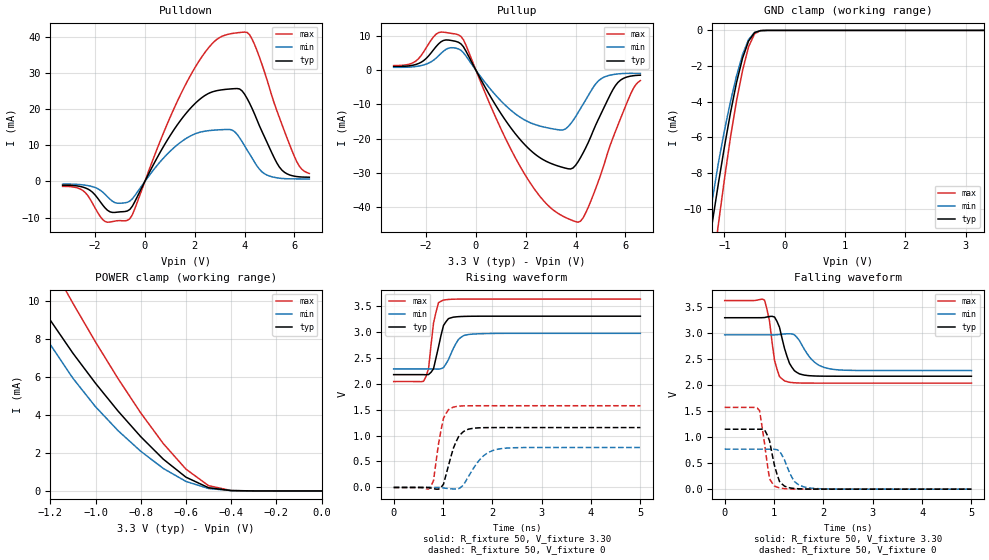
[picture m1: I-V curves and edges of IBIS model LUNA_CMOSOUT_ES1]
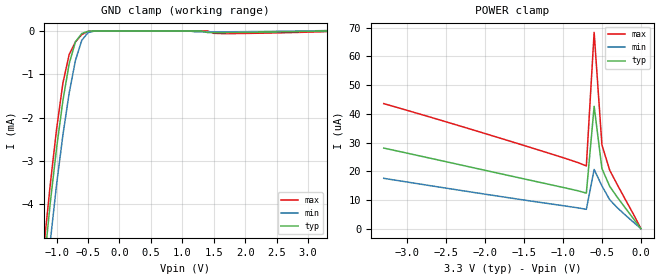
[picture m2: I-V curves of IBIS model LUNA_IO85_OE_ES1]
[IBIS Ver]   3.2
[Comment Char]   |_char
[File name]   sg-9101cx_33v_a.ibs
[File Rev]   1.0
[Date]   2017/11/24 15:54:02
[Source]
[Notes]
[Disclaimer]
This information is for modeling purposes only, and is not guaranteed.
Property of SEIKO EPSON Corp.,
unauthorized reproduction and/or distribution is strictly prohibited.
[Copyright]
Copyright 2017, SEIKO EPSON Corp.
[Component]   SG-9101CA
Si_location Pin
Timing_location Pin
[Manufacturer]   SEIKO EPSON Corp.
| 7050 PKG
| 7050 PKG
[Package]
R_pkg   224m   NA   NA
L_pkg   5.5n   NA   NA
C_pkg   0.144p   NA   NA
[Pin] signal_name   model_name
1   OE   LUNA_IO85_OE_ES1
2   VSS   GND
3   OUT   LUNA_CMOSOUT_ES1
4   VDD   POWER
[Component]   SG-9101CB
Si_location Pin
Timing_location Pin
[Manufacturer]   SEIKO EPSON Corp.
| 5032 PKG
| 5032 PKG
[Package]
R_pkg   200m   NA   NA
L_pkg   2.16n   NA   NA
C_pkg   1.23p   NA   NA
[Pin] signal_name   model_name
1   OE   LUNA_IO85_OE_ES1
2   VSS   GND
3   OUT   LUNA_CMOSOUT_ES1
4   VDD   POWER
[Component]   SG-9101CE
Si_location Pin
Timing_location Pin
[Manufacturer]   SEIKO EPSON Corp.
| 3225 PKG
| 3225 PKG
[Package]
R_pkg   177m   NA   NA
L_pkg   4.5n   NA   NA
C_pkg   0.64p   NA   NA
[Pin] signal_name   model_name
1   OE   LUNA_IO85_OE_ES1
2   VSS   GND
3   OUT   LUNA_CMOSOUT_ES1
4   VDD   POWER
[Component]   SG-9101CG
Si_location Pin
Timing_location Pin
[Manufacturer]   SEIKO EPSON Corp.
| 2520 PKG
| 2520 PKG
[Package]
R_pkg   238m   NA   NA
L_pkg   2.1n   NA   NA
C_pkg   0.38p   NA   NA
[Pin] signal_name   model_name
1   OE   LUNA_IO85_OE_ES1
2   VSS   GND
3   OUT   LUNA_CMOSOUT_ES1
4   VDD   POWER
| Models and submodels in the file (2): LUNA_CMOSOUT_ES1 (3-state), LUNA_IO85_OE_ES1 (Input)
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[Model]   LUNA_CMOSOUT_ES1
Model_type 3-state
Enable Active-High
Polarity Non-Inverting
Vmeas=1.65
C_comp   2.5p   2.0p   3.0p
[Temperature Range] 25   105   -40
[Voltage Range]   3.30   2.97   3.63
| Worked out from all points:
|   slope of the pulldown table from 0 to 0.495 V, typ, clamps not added: 75.2 ohm
|   slope of the pullup table from 0 to 0.495 V, typ, clamps not added: 75.3 ohm
|   GND clamp passes 1 mA (typ) near -0.64 V on its own axis
|   POWER clamp passes 1 mA (typ) near -0.63 V on its own axis
|   falling waveform, R_fixture 50, V_fixture 3.30: 20-80 % time 207ps typ, 322ps min, 155ps max; typ from 3.3 V to 2.17 V
|   falling waveform, R_fixture 50, V_fixture 0: 20-80 % time 170ps typ, 227ps min, 143ps max; typ from 1.15 V to 0 V
|   rising waveform, R_fixture 50, V_fixture 3.30: 20-80 % time 163ps typ, 216ps min, 127ps max; typ from 2.17 V to 3.3 V
|   rising waveform, R_fixture 50, V_fixture 0: 20-80 % time 230ps typ, 348ps min, 160ps max; typ from 0 V to 1.15 V
[Pullup]
-3.3V     1.06mA     815.2uA    1.324mA
-2.4V     1.678mA    1.074mA    2.704mA
-1.5V     7.647mA    4.171mA    10.95mA
-600mV    7.664mA    5.788mA    9.824mA
900mV     -11.47mA   -8.159mA   -15.48mA
2.1V      -22.76mA   -15.07mA   -32mA
3.5V      -28.4mA    -17.44mA   -42.63mA
4.1V      -26.71mA   -12.39mA   -44.35mA
4.9V      -14.57mA   -3.238mA   -32.71mA
5.6V      -4.486mA   -1.181mA   -17.87mA
6.3V      -1.64mA    -938.9uA   -5.579mA
6.6V      -1.468mA   -942.3uA   -3.051mA
[Pulldown]
-3.3V     -1.038mA   -736.1uA   -1.359mA
-2.4V     -1.756mA   -1.02mA    -3.001mA
-1.6V     -7.274mA   -3.52mA    -11.03mA
-600mV    -7.7mA     -5.412mA   -10.26mA
1V        12.51mA    8.249mA    17.5mA
2.1V      22.07mA    13.36mA    32.44mA
3.5V      25.58mA    14.21mA    40.86mA
4V        24.11mA    9.852mA    41.25mA
4.4V      18.66mA    5.363mA    37.85mA
5.4V      3.963mA    903.3uA    17.62mA
6.1V      1.352mA    712.3uA    5.408mA
6.6V      1.173mA    678.8uA    2.205mA
[GND Clamp]
-3.3V     -86.74mA   -76.76mA   -101.8mA
-1.3V     -13.11mA   -11.85mA   -16.24mA
-1.2V     -10.77mA   -9.503mA   -13.52mA
-1.1V     -8.591mA   -7.44mA    -10.88mA
-1V       -6.541mA   -5.623mA   -8.358mA
-900mV    -4.635mA   -4.001mA   -6.009mA
-800mV    -2.939mA   -2.563mA   -3.961mA
-700mV    -1.565mA   -1.365mA   -2.263mA
-600mV    -601.2uA   -521.6uA   -925.2uA
-500mV    -121.4uA   -116.4uA   -188.8uA
-300mV    -500.8nA   -1.29uA    -313.6nA
3.3V      193.1pA    4.095uA    131.4pA
[POWER Clamp]
-3.3V     73.68mA    63.39mA    89.04mA
-1.4V     13.2mA     11.93mA    16.56mA
-1.3V     10.93mA    9.714mA    14.21mA
-1.2V     8.97mA     7.69mA     11.99mA
-1.1V     7.236mA    5.92mA     9.861mA
-1V       5.655mA    4.424mA    7.824mA
-900mV    4.191mA    3.162mA    5.894mA
-700mV    1.665mA    1.179mA    2.483mA
-600mV    721.7uA    498.7uA    1.143mA
-500mV    167.2uA    126.9uA    275.1uA
-400mV    16.41uA    18.75uA    19.76uA
0V        193.1pA    1.068nA    160pA
[Falling Waveform]
R_fixture=50
V_fixture=3.30
V_fixture_min=2.97
V_fixture_max=3.63
0s        3.3V       2.97V      3.63V
808.1ps   3.304V     2.97V      3.639V
909.1ps   3.324V     2.97V      3.23V
1.01ns    3.313V     2.97V      2.478V
1.111ns   3.115V     2.978V     2.167V
1.212ns   2.71V      2.988V     2.085V
1.465ns   2.246V     2.921V     2.045V
1.818ns   2.179V     2.446V     2.041V
2.121ns   2.175V     2.318V     2.041V
5ns       2.174V     2.284V     2.041V
[Falling Waveform]
R_fixture=50
V_fixture=0
V_fixture_min=0
V_fixture_max=0
0s        1.154V     769.7mV    1.574V
606.1ps   1.154V     769.7mV    1.573V
707.1ps   1.154V     769.7mV    1.512V
808.1ps   1.141V     769.7mV    877.7mV
909.1ps   929.1mV    769.5mV    198.4mV
1.01ns    450.2mV    769.2mV    59.15mV
1.111ns   147.4mV    734.1mV    23.18mV
1.414ns   12.74mV    146.6mV    1.885mV
1.667ns   2.536mV    31.77mV    214.1uV
5ns       0V         0V         0V
[Rising Waveform]
R_fixture=50
V_fixture=3.30
V_fixture_min=2.97
V_fixture_max=3.63
0s        2.174V     2.284V     2.041V
606.1ps   2.174V     2.284V     2.046V
707.1ps   2.176V     2.284V     2.287V
808.1ps   2.288V     2.284V     3.168V
909.1ps   2.709V     2.28V      3.56V
1.01ns    3.121V     2.309V     3.611V
1.111ns   3.253V     2.464V     3.623V
1.313ns   3.291V     2.851V     3.629V
1.515ns   3.298V     2.947V     3.63V
5ns       3.3V       2.97V      3.63V
[Rising Waveform]
R_fixture=50
V_fixture=0
V_fixture_min=0
V_fixture_max=0
0s        0V         0V         0V
757.6ps   -13.16mV   -37.66uV   26.8mV
808.1ps   -24.61mV   51.13uV    132.7mV
909.1ps   -33.13mV   506.3uV    836.1mV
1.01ns    62.11mV    -9.902mV   1.334V
1.212ns   760.5mV    -29.26mV   1.548V
1.465ns   1.102V     126.8mV    1.573V
1.818ns   1.152V     607.4mV    1.574V
2.121ns   1.154V     739.2mV    1.574V
5ns       1.154V     769.7mV    1.574V
[Ramp]
R_load=50
dV/dt_r   6.923E-1/2.262E-10   4.618E-1/3.482E-10   9.446E-1/1.556E-10
dV/dt_f   6.756E-1/2.073E-10   4.116E-1/3.220E-10   9.534E-1/1.485E-10
|[End   LUNA_CMOSOUT_ES1
[Model]   LUNA_IO85_OE_ES1
Model_type Input
Enable Active-Low
Polarity Non-Inverting
Vinh=2.55
Vinl=0.89
C_comp   2.5p   2.0p   3.0p
[Temperature Range] 25   105   -40
[Voltage Range]   3.30   2.97   3.63
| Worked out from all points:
|   GND clamp passes 1 mA (typ) near -0.83 V on its own axis
[GND Clamp]
-3.3V     -49.97mA   -47.74mA   -53.94mA
-1.2V     -5.408mA   -6.351mA   -4.953mA
-1.1V     -3.959mA   -4.854mA   -3.533mA
-1V       -2.702mA   -3.543mA   -2.264mA
-900mV    -1.612mA   -2.406mA   -1.207mA
-800mV    -755.8uA   -1.435mA   -544.3uA
-700mV    -251.9uA   -680.1uA   -254.3uA
-600mV    -60.6uA    -218.5uA   -85.08uA
-500mV    -8.506uA   -39.85uA   -10.99uA
-400mV    -1.005uA   -4.241uA   -1.145uA
1.7V      -37.51uA   -20.16uA   -61.79uA
3.3V      135.9pA    8.008uA    -15.73uA
[POWER Clamp]
-3.3V     28.08uA    17.53uA    43.56uA
-1.6V     17.94uA    10.38uA    29.81uA
-900mV    13.77uA    7.613uA    23.86uA
-700mV    12.37uA    6.737uA    21.84uA
-600mV    42.62uA    20.63uA    68.38uA
-500mV    20.91uA    14.89uA    29.15uA
-400mV    14.72uA    10.06uA    20.36uA
-300mV    10.84uA    7.224uA    15.17uA
-100mV    3.62uA     2.354uA    5.264uA
0V        135.7pA    303.7pA    135.4pA
